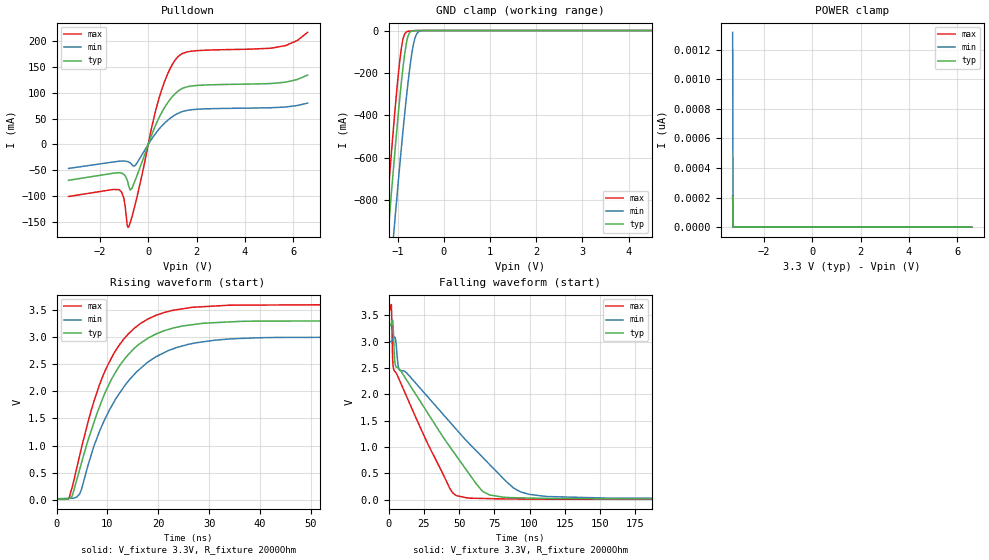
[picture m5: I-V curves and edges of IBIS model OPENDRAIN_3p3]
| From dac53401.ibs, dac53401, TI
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|   OPENDRAIN_3p3 Model
[Model]   OPENDRAIN_3p3
Model_type   I/O_open_drain
Polarity   Non-Inverting
Enable   Active-Low
Vinl = 0.4
Vinh = 1.62
Vmeas = 1.65
Vref = 3.3
Cref = 2pF
Rref = 2000
|   typ   min   max
C_comp   1.131pF   1.106pF   1.153pF
[Voltage Range]   3.3   3   3.6
[Temperature Range]   25   125   -40
[Pullup Reference]   3.3   3   3.6
[Pulldown Reference]   0   -0   0
[Power Clamp Reference]   3.3   3   3.6
[GND Clamp Reference]   0   0   0
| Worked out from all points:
|   slope of the pulldown table from 0 to 0.495 V, typ, clamps not added: 8.87 ohm
|   GND clamp passes 1 mA (typ) near -0.66 V on its own axis
|   falling waveform, V_fixture 3.3V, R_fixture 2000Ohm: 20-80 % time 48.1ns typ, 60.7ns min, 31.5ns max; typ from 3.3 V to 0.012 V
|   rising waveform, V_fixture 3.3V, R_fixture 2000Ohm: 20-80 % time 8.9ns typ, 10.2ns min, 8.24ns max; typ from 0.012 V to 3.3 V
[Pulldown]
|   Voltage   I(typ)   I(min)   I(max)
-3.3V     -69.1mA    -46.26mA   -100.3mA
-1.191V   -54.48mA   -32.27mA   -87.74mA
-1.013V   -57.52mA   -31.89mA   -103.3mA
-874.5mV  -67.87mA   -32.75mA   -153.5mA
-815.1mV  -78.37mA   -33.62mA   -159.4mA
-745.8mV  -87.88mA   -35.39mA   -151mA
-537.9mV  -68.99mA   -40.46mA   -115.3mA
432.3mV   50.04mA    28.78mA    86.43mA
848.1mV   83.21mA    48.26mA    140.4mA
1.195V    101.2mA    59.03mA    167.3mA
5.669V    119.9mA    72.15mA    190.4mA
6.6V      133.8mA    79.76mA    216.2mA
[GND Clamp]
|   Voltage   I(typ)   I(min)   I(max)
-3.3V     -6.897A    -6.981A    -6.923A
-1.33V    -1.28A     -1.584A    -1.107A
-1.241V   -1.037A    -1.35A     -855.9mA
-1.211V   -957mA     -1.272A    -773.2mA
-1.142V   -772.7mA   -1.093A    -583.9mA
-1.063V   -568.5mA   -891.7mA   -377.7mA
-924mV    -244.9mA   -555.3mA   -84.05mA
-884.4mV  -166.7mA   -465.1mA   -36.27mA
-805.2mV  -48.92mA   -296.7mA   -5.651mA
-656.7mV  -831uA     -60.15mA   -749.1uA
-498.3mV  -21.67uA   -1.403mA   -21.19uA
6.6V      0A         0A         0A
[POWER Clamp]
|   Voltage   I(typ)   I(min)   I(max)
-3.3V     204.8pA    1.318nA    216pA
-3.28V    0A         0A         0A
-3.27V    0A         0A         0A
6.6V      0A         0A         0A
[Ramp]
R_load = 2000
|   typ   min   max
dV/dt_r   1.97274/8.89396e-09   1.78838/1.01436e-08   2.15555/8.24733e-09
dV/dt_f   1.97274/4.8229e-08   1.78837/6.07015e-08   2.15555/3.13876e-08
[Falling Waveform]
V_fixture = 3.3V
V_fixture_min = 3V
V_fixture_max = 3.6V
R_fixture = 2000Ohm
C_fixture = 0F
|   Time   V(typ)   V(min)   V(max)
0s        3.3V       3V         3.6V
1.935ns   3.349V     3.002V     3.699V
2.844ns   3.401V     3.038V     2.691V
3.754ns   2.936V     3.077V     2.462V
7.721ns   2.475V     2.456V     2.267V
43.22ns   1.014V     1.481V     227.2mV
56.02ns   532.9mV    1.098V     33.18mV
71.61ns   90.54mV    670.1mV    21.03mV
113.6ns   22.92mV    59.8mV     11.7mV
1.5us     12.11mV    19.38mV    7.413mV
[Rising Waveform]
V_fixture = 3.3V
V_fixture_min = 3V
V_fixture_max = 3.6V
R_fixture = 2000Ohm
C_fixture = 0F
|   Time   V(typ)   V(min)   V(max)
0s        12.1mV     19.37mV    7.412mV
2.481ns   22.89mV    25.66mV    40.06mV
3.1ns     77.53mV    27.23mV    241mV
4.531ns   552.1mV    105mV      808mV
6.829ns   1.276V     829.7mV    1.65V
8.915ns   1.828V     1.362V     2.234V
14.13ns   2.678V     2.19V      3.059V
21.81ns   3.135V     2.743V     3.468V
33.88ns   3.278V     2.963V     3.587V
1.5us     3.3V       3V         3.6V
